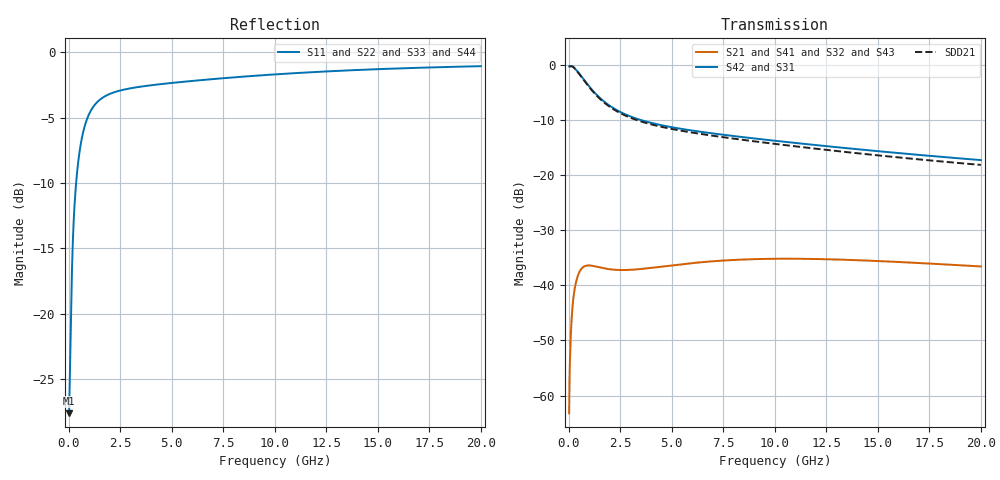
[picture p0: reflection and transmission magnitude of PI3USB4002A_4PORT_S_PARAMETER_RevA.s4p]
! Created Fri Sep 13 09:37:11 2024
# hz S ma R 50
! 4 Port Network Data from SP1.SP block
! freq  magS11  angS11  magS12  angS12  magS13  angS13  magS14  angS14
!  magS21  angS21  magS22  angS22  magS23  angS23  magS24  angS24
!  magS31  angS31  magS32  angS32  magS33  angS33  magS34  angS34
!  magS41  angS41  magS42  angS42  magS43  angS43  magS44  angS44
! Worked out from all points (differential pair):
!   1000 points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, 20 MHz to 20 GHz, reference 50 ohm
!   strongest paths, dB at 20 MHz, 5.02 GHz, 10.02 GHz, 15.02 GHz, 20 GHz:
!     S42: -0.3, -11.4, -13.8, -15.7, -17.3
!     S31: -0.3, -11.4, -13.8, -15.7, -17.3
!     S21: -63.2, -36.4, -35.2, -35.6, -36.6
!     S41: -63.2, -36.4, -35.2, -35.6, -36.6
!     S32: -63.2, -36.4, -35.2, -35.6, -36.6
!     S43: -63.2, -36.4, -35.2, -35.6, -36.6
!   taken as a pair (ports 2,1 in; 4,3 out), SDD21 dB: -0.3, -11.7, -14.4, -16.5, -18.2
!   lowest |S11| = -27.6 dB at 20 MHz (marker M1), VSWR 1.09, Z = 54 - j1.75 ohm
!   |S11| at or under -10 dB: start of sweep to 359.2 MHz
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2e7  0.04172 -22.8  0.0006914 88.1  0.9617 -1.0  0.0006913 88.1
     0.0006914 88.1  0.04172 -22.8  0.0006913 88.1  0.9617 -1.0
     0.9617 -1.0  0.0006913 88.1  0.04185 -23.4  0.0006913 88.1
     0.0006913 88.1  0.9617 -1.0  0.0006913 88.1  0.04185 -23.4
1.6e8  0.1489 -77.5  0.005569 73.1  0.9648 -8.7  0.005561 73.1
       0.005569 73.1  0.1489 -77.5  0.005561 73.1  0.9648 -8.7
       0.9648 -8.7  0.005561 73.1  0.1494 -78.8  0.005552 73.0
       0.005561 73.1  0.9648 -8.7  0.005552 73.0  0.1494 -78.8
2.8e8  0.2582 -96.6  0.00903 58.9  0.9282 -16.0  0.009015 58.9
       0.00903 58.9  0.2582 -96.6  0.009015 58.9  0.9282 -16.0
       0.9282 -16.0  0.009015 58.9  0.2573 -97.2  0.009001 58.9
       0.009015 58.9  0.9282 -16.0  0.009001 58.9  0.2573 -97.2
8.4e8  0.5415 -132.3  0.01502 21.2  0.6874 -35.7  0.01501 21.2
       0.01502 21.2  0.5415 -132.3  0.01501 21.2  0.6874 -35.7
       0.6874 -35.7  0.01501 21.2  0.5413 -132.4  0.015 21.2
       0.01501 21.2  0.6874 -35.7  0.015 21.2  0.5413 -132.4
1.8e9  0.6812 -152.6  0.01413 4.9  0.4488 -44.6  0.01412 5.0
       0.01413 4.9  0.6812 -152.6  0.01412 5.0  0.4488 -44.6
       0.4488 -44.6  0.01412 5.0  0.6814 -152.7  0.01411 5.0
       0.01412 5.0  0.4488 -44.6  0.01411 5.0  0.6814 -152.7
3.72e9  0.7426 -163.5  0.01417 3.9  0.3055 -45.6  0.01416 3.9
        0.01417 3.9  0.7426 -163.5  0.01416 3.9  0.3055 -45.6
        0.3055 -45.6  0.01416 3.9  0.7428 -163.5  0.01416 3.9
        0.01416 3.9  0.3055 -45.6  0.01416 3.9  0.7428 -163.5
2e10  0.8841 -175.1  0.0148 -44.9  0.1361 -71.5  0.01476 -44.8
      0.0148 -44.9  0.8841 -175.1  0.01476 -44.8  0.1361 -71.5
      0.1361 -71.5  0.01476 -44.8  0.8843 -175.1  0.01478 -45.0
      0.01476 -44.8  0.1361 -71.5  0.01478 -45.0  0.8843 -175.1
